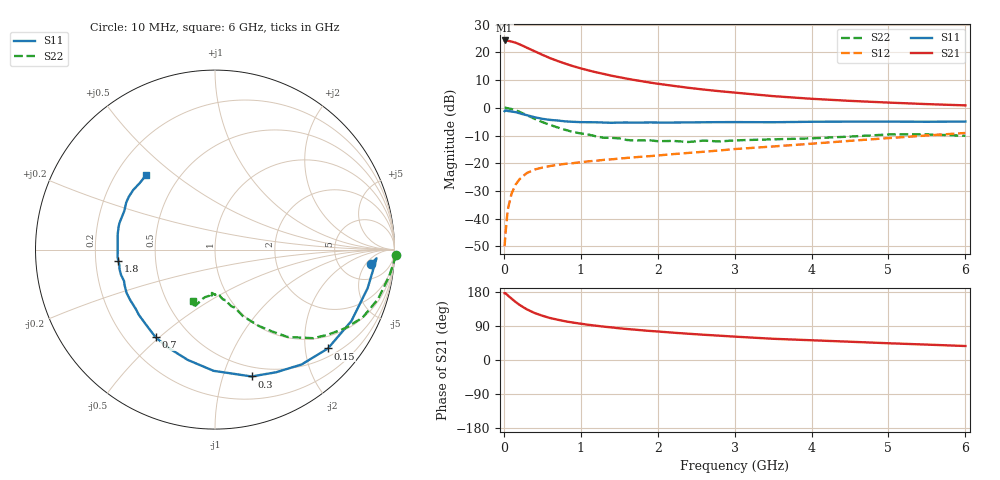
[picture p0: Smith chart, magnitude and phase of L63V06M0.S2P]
!  INFINEON TECHNOLOGIES Small Signal Semiconductors
! BFR380L3 , Si-NPN RF-Transistor in TSLP-3-1
!  Vce=3 V,  Ic=6 mA
! Common Emitter S-Parameters:  07. March 2005
#  GHz  S  MA  R  50
! f  S11  S21  S12  S22
! GHz  Mag  Ang  Mag  Ang  Mag  Ang  Mag  Ang
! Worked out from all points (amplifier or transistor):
!   36 points, 10 MHz to 6 GHz, reference 50 ohm
!   highest |S21| = 24.3 dB at 10 MHz (marker M1)
!   |S21| within 3 dB of that: start of sweep to 329.5 MHz
!   unconditionally stable (mu >= 1): 2.316 GHz to 4.708 GHz
!   at 250 MHz: K = 0.19, MSG = 23.5 dB, |S12| = -24.6 dB
!   at 1.4 GHz: K = 0.80, MSG = 15.1 dB, |S12| = -18.6 dB
!   at 6 GHz: K = 0.94, MSG = 5.0 dB, |S12| = -9.1 dB
!   S11 on the Smith chart (normalised r, x): 10 MHz: 10, -7; 150 MHz: 0.68, -2.50; 300 MHz: 0.40, -1.25; 700 MHz: 0.32, -0.49; 1.8 GHz: 0.30, -0.05; 6 GHz: 0.33, +0.40
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0.01  0.8707 -5.3  16.38 176.4  0.0032 81.8  1.011 -1.8
0.02  0.9014 -3.1  16.26 176.5  0.0051 87.7  1 -3.7
0.05  0.8771 -14.2  16.19 170.7  0.0144 85.1  0.9821 -8.6
0.1  0.8578 -27.6  15.65 162.0  0.0283 76.9  0.9498 -16.8
0.15  0.8363 -41.2  14.96 153.6  0.0406 69.1  0.9054 -24.7
0.2  0.8015 -53.0  14.03 146.0  0.0507 64.6  0.8507 -30.8
0.25  0.7636 -63.5  13.07 139.7  0.0589 59.9  0.7891 -36.9
0.3  0.7357 -73.9  12.11 133.6  0.0667 56.0  0.7376 -42.0
0.4  0.6754 -90.7  10.46 124.0  0.077 50.5  0.6326 -50.3
0.5  0.633 -103.9  9.038 116.9  0.0836 47.0  0.5531 -55.3
0.6  0.6055 -115.4  7.876 110.8  0.0891 44.4  0.4921 -60.0
0.7  0.5901 -124.1  6.979 106.3  0.0937 43.8  0.441 -63.7
0.9  0.5589 -139.3  5.634 98.7  0.1004 42.8  0.3644 -69.5
1.1  0.5498 -149.1  4.727 92.9  0.1083 43.7  0.3294 -73.8
1.4  0.5362 -161.0  3.789 86.0  0.1177 45.3  0.2875 -78.5
1.8  0.5422 -173.5  3.007 78.3  0.1315 48.5  0.258 -84.9
2.2  0.5424 178.0  2.492 72.1  0.1462 51.3  0.2529 -89.5
2.8  0.5516 166.9  1.996 64.2  0.17 55.4  0.2469 -97.2
3.5  0.5494 156.8  1.624 56.0  0.2009 57.5  0.2702 -101.7
4.5  0.5633 148.5  1.334 48.2  0.2537 60.6  0.303 -106.5
5.5  0.5596 138.7  1.166 40.6  0.3167 60.3  0.3313 -111.0
6  0.5652 132.9  1.106 36.9  0.3518 59.2  0.3129 -113.3
